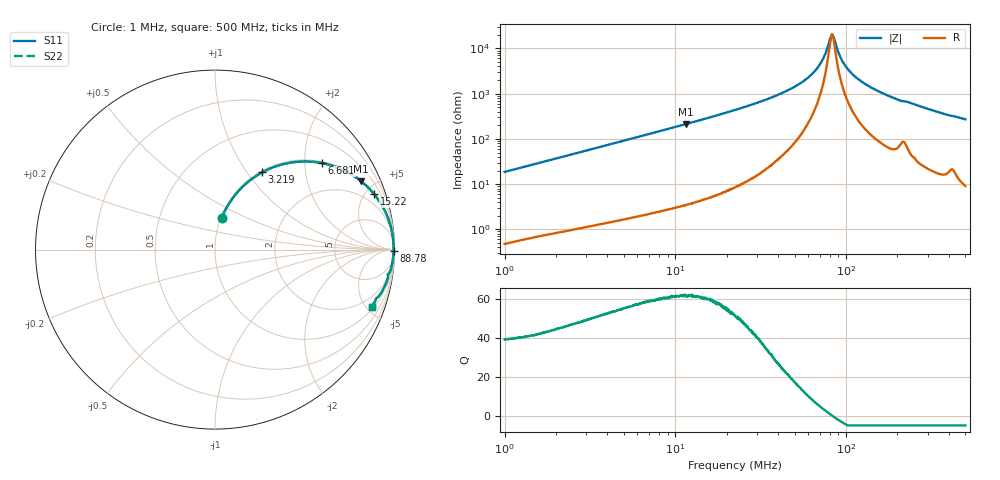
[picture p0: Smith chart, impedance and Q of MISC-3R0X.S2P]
!s-Parameter Generated by FASTRON Sdn. Bhd.
!FASTRON P/N : MISC-3R0X
!Keysight Technologies,E4991B,MY54100416,A.01.15
!Date: Mon Mar 16 10:30:46 2026
!Version  : Rev00 Mon Mar 16 10:30:46 2026
!Data & Calibration Information:
!PortZ  Port1:50+j0  Port2:50+j0
!When reading, reference impedance value at option line is always used.
!Remarks : This data is being provided solely for informational purposes.
!Freq	S11	S21	S12	S22
# Hz S dB R 50
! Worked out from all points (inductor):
!   1601 points, 1 MHz to 500 MHz, reference 50 ohm
!   read as one part in series: L = 2.95 uH near 1.032 MHz
!   highest Q = 61.5 at 11.51 MHz (marker M1), where L = 2.94 uH
!   self-resonance near 82.79 MHz
!   S11 on the Smith chart (normalised r, x): 1 MHz: 1.01, +0.37; 3.219 MHz: 1.02, +1.18; 6.681 MHz: 1.04, +2.45; 15.22 MHz: 1.10, +5.70; 88.78 MHz: open; 500 MHz: 1.18, -5.42
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1000000  -14.77 78.0  -0.19 -10.5  -0.19 -10.5  -14.77 78.0
1763117  -10.24 70.8  -0.50 -17.9  -0.50 -17.9  -10.24 70.8
2820919  -6.81 61.7  -1.11 -27.1  -1.11 -27.1  -6.81 61.7
3219169  -5.95 58.6  -1.38 -30.3  -1.38 -30.3  -5.95 58.6
6681481  -2.29 38.9  -4.05 -50.1  -4.05 -50.1  -2.29 38.9
7957584  -1.74 34.1  -5.02 -54.9  -5.02 -54.9  -1.74 34.1
1.150887e7  -0.92 25.0  -7.48 -64.1  -7.48 -64.1  -0.92 25.0
1.522251e7  -0.55 19.2  -9.65 -69.8  -9.65 -69.8  -0.55 19.2
2.236068e7  -0.26 12.9  -13.06 -76.0  -13.06 -76.0  -0.26 12.9
4.327634e7  -0.07 5.3  -20.73 -82.3  -20.73 -82.3  -0.07 5.3
5.379161e7  -0.05 3.4  -24.58 -82.6  -24.58 -82.6  -0.05 3.4
6.307767e7  -0.04 2.1  -28.68 -81.0  -28.68 -81.0  -0.04 2.1
7.254416e7  -0.04 1.0  -34.77 -74.3  -34.77 -74.3  -0.04 1.0
8.214513e7  -0.04 0.1  -46.01 -14.3  -46.01 -14.3  -0.04 0.1
8.47377e7  -0.04 -0.2  -44.87 30.2  -44.87 30.2  -0.04 -0.2
8.878078e7  -0.04 -0.5  -39.73 60.2  -39.73 60.2  -0.04 -0.5
9.745486e7  -0.05 -1.2  -33.15 74.8  -33.15 74.8  -0.05 -1.2
1.112133e8  -0.06 -2.2  -28.07 79.6  -28.07 79.6  -0.06 -2.2
1.350515e8  -0.07 -3.8  -23.51 80.8  -23.51 80.8  -0.07 -3.8
1.77937e8  -0.12 -6.3  -19.12 79.6  -19.12 79.6  -0.12 -6.3
3.497673e8  -0.37 -14.3  -12.13 73.2  -12.13 73.2  -0.37 -14.3
5e8  -0.65 -20.0  -9.32 68.1  -9.32 68.1  -0.65 -20.0
